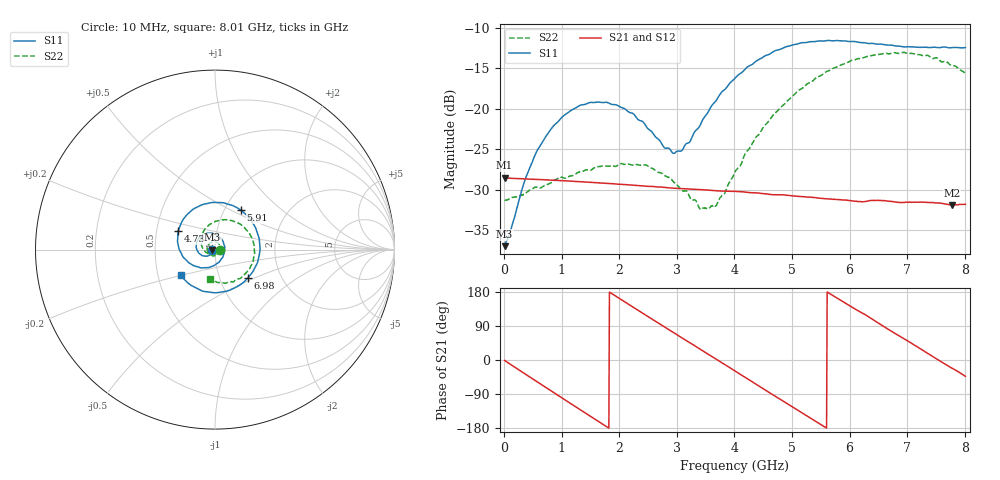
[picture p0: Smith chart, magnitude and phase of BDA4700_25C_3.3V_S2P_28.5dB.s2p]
!Agilent Technologies,E5071B,MY42404982,A.09.10
!Date: Mon Oct 20 18:15:03 2025
!Data & Calibration Information:
!Freq	S11:SOLT2(ON)	S21:SOLT2(ON)	S12:SOLT2(ON)	S22:SOLT2(ON)
# Hz S RI R 50
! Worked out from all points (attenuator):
!   801 points, 10 MHz to 8.01 GHz, reference 50 ohm
!   highest |S21| = -28.54 dB at 10 MHz (marker M1); lowest = -31.9 dB at 7.78 GHz (marker M2)
!   lowest |S11| = -37.0 dB at 10 MHz (marker M3), VSWR 1.03, Z = 48.6 - j0.126 ohm
!   |S11| at or under -10 dB: start of sweep to end of sweep
!   |S22| runs from -32.5 to -13.0 dB; largest |S21 - S12| = 0.00049
!   S11 on the Smith chart (normalised r, x): 10 MHz: 0.97, -0.00; 4.73 GHz: 0.65, +0.14; 5.91 GHz: 1.19, +0.56; 6.98 GHz: 1.36, -0.45; 8.01 GHz: 0.65, -0.20
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1e7  -0.0141 -0.0013  0.0374 -0.000769  0.0373 -0.000834  0.0271 -0.000831
3.6e8  -0.0247 -0.0261  0.0297 -0.0218  0.0297 -0.0218  0.0227 -0.0191
5.8e8  -0.0422 -0.0361  0.0194 -0.031  0.0194 -0.031  0.0145 -0.0292
1e9  -0.0847 -0.0243  -0.00591 -0.0354  -0.00592 -0.0354  -0.0146 -0.0348
1.35e9  -0.105 0.0137  -0.0244 -0.0255  -0.0245 -0.0255  -0.0365 -0.0183
1.97e9  -0.0592 0.0867  -0.0331 0.00844  -0.0331 0.00846  -0.0349 0.0277
2.45e9  0.0159 0.078  -0.0163 0.0289  -0.0163 0.029  -0.00359 0.0448
2.68e9  0.0439 0.0478  -0.00419 0.0325  -0.00423 0.0325  0.0127 0.0384
2.93e9  0.0531 0.00334  0.00914 0.031  0.00912 0.0309  0.0249 0.0255
3.06e9  0.0502 -0.0216  0.0156 0.0281  0.0152 0.0282  0.0278 0.0157
3.44e9  0.00203 -0.0842  0.0286 0.0134  0.0286 0.0134  0.0198 -0.0136
3.69e9  -0.0521 -0.1008  0.0311 0.000815  0.0311 0.000744  0.00166 -0.0252
4.01e9  -0.1307 -0.0824  0.027 -0.0149  0.027 -0.0148  -0.031 -0.026
4.73e9  -0.2049 0.1048  -0.00383 -0.0291  -0.00366 -0.0291  -0.0789 0.054
5.35e9  -0.0597 0.2533  -0.0259 -0.0113  -0.0259 -0.0115  -0.0159 0.1467
5.91e9  0.1432 0.221  -0.0239 0.013  -0.0239 0.0129  0.1089 0.1556
6.29e9  0.2322 0.105  -0.0125 0.0236  -0.0122 0.0236  0.1861 0.0976
6.68e9  0.2424 -0.0507  0.0046 0.0264  0.00469 0.0264  0.2191 0.000729
6.98e9  0.1835 -0.1572  0.0159 0.0211  0.0159 0.021  0.2065 -0.0788
7.41e9  0.0281 -0.2376  0.0256 0.00564  0.0257 0.00564  0.1272 -0.1634
7.78e9  -0.1219 -0.2056  0.0235 -0.00948  0.0236 -0.00947  0.0258 -0.1832
8.01e9  -0.1914 -0.1441  0.0187 -0.0175  0.0188 -0.0174  -0.0295 -0.1635
